PROGRAM MAIN_Slow
VAR CONSTANT
	cInitOrderSpec : ST_CM_OrderPowerSpectrum_InitPars := (	fSampleRateVibration	:= cSampleRateVib, 
															fSampleRatePosition		:= cSampleRatePos, 
															fPositionScaling		:= cShaftPerimeter, 
															fMaxRPM					:= cMaxRPM, 
															nFFT_Length				:= cFFTLength , 
															nWindowLength			:= cWindowLength, 	
															bTransformToDecibel		:= FALSE, 
															eWindowType				:= E_CM_WindowType.eCM_HannWindow,
															eScalingType			:= E_CM_ScalingType.eCM_PowerSpectralDensity );
	cInitPowerSpec : ST_CM_PowerSpectrum_InitPars := (		nFFT_Length				:= cFFTLength , 
															nWindowLength			:= cWindowLength, 	
															bTransformToDecibel		:= FALSE, 
															eWindowType				:= E_CM_WindowType.eCM_HannWindow,
															eScalingType			:= E_CM_ScalingType.eCM_PowerSpectralDensity );
END_VAR
VAR
	fbOrderSpec		: FB_CMA_OrderPowerSpectrum :=(	stInitPars := cInitOrderSpec, nOwnID := eID_OrderSpec, aDestIDs := [eID_Sink_OrderSpec] );	
	fbPowerSpec		: FB_CMA_PowerSpectrum :=(	stInitPars := cInitPowerSpec, nOwnID := eID_PwrSpec, aDestIDs := [eID_Sink_PwrSpec] );	
	
	fbErrHist		: FB_HRErrHist; // error monitoring
END_VAR

// Call OrderPowerSpectrum
fbOrderSpec.Call();
IF fbOrderSpec.bError THEN
	fbErrHist.AddError(bErr:=TRUE, hrErrCode:=fbOrderSpec.hrErrorCode, sErrSource:='MAIN_Slow.fbOrderSpec.Call()'); // error monitoring
	// ToDo: if error
END_IF

// Call PowerSpectrum	
fbPowerSpec.Call();
IF fbPowerSpec.bError THEN
	fbErrHist.AddError(bErr:=TRUE, hrErrCode:=fbOrderSpec.hrErrorCode, sErrSource:='MAIN_Slow.fbPowerSpec.Call()'); // error monitoring
	// ToDo: if error
END_IF

END_PROGRAM
